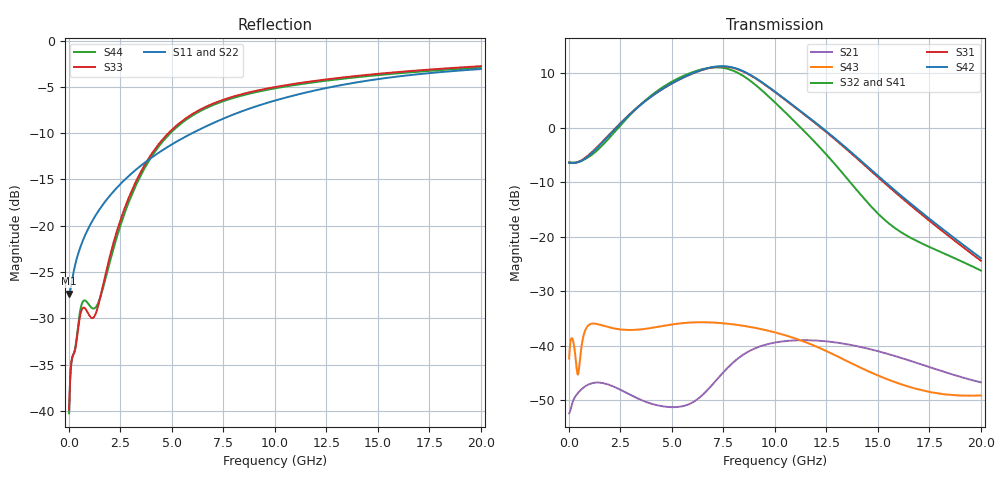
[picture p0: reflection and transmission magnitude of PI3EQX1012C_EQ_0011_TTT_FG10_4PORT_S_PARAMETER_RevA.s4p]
! NPort=4 DATA=2000 NOISE=0 GROUPDELAY=0 COMPLEX_DATAFORMAT=POLAR
! NumOfBlock=1 NumOfParam=0
! .MODEL Smodel S TSTONEFILE=PI3EQX1012C_EQ_0011_TTT_FG10_4PORT_S_PARAMETER_RevA.s4p TYPE=S
!  -- The above .MODEL line can be used for the S element in the netlist.
! The s parameter is extracted from the linear redriver, it is not bi-directional; only s(4,1)s(4,2) and s(3,1)s(3,2)
! should be the insertion loss
!Port definition:
!Port1 = input+
!Port2 = input-
!Port3 = output+
!Port4 = output-
# Hz S MA R  50
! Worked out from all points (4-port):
!   2000 points, 10 MHz to 20 GHz, reference 50 ohm
!   strongest paths, dB at 10 MHz, 5.01 GHz, 10.01 GHz, 15.01 GHz, 20 GHz:
!     S42: -6.4, 8.1, 6.6, -8.9, -24.0
!     S31: -6.4, 8.1, 6.5, -9.1, -24.4
!     S32: -6.4, 8.5, 4.6, -15.8, -26.2
!     S41: -6.4, 8.5, 4.7, -16.0, -26.6
!     S43: -42.4, -36.1, -37.6, -45.5, -49.2
!     S21: -52.4, -51.3, -39.5, -41.0, -46.8
!   lowest |S11| = -27.3 dB at 10 MHz (marker M1), VSWR 1.09, Z = 45.9 - j0.123 ohm
!   |S11| at or under -10 dB: start of sweep to 5.987 GHz
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1e7  0.04301 -178.2  0.002379 1.5  0.0008102 -0.5  0.0008039 -0.5
     0.002388 1.5  0.04109 -178.1  0.000927 -0.5  0.0009197 -0.5
     0.4783 -0.3  0.4774 179.8  0.01016 -4.0  0.007598 -25.7
     0.4769 179.8  0.4792 -0.3  0.007615 -25.8  0.009722 -4.1
4.07e9  0.2357 -124.4  0.002943 -0.6  0.0003837 -56.7  0.0003819 -57.1
        0.0029 -0.5  0.2393 -123.3  0.0004361 -57.4  0.0004341 -57.8
        1.973 -64.8  2.021 127.6  0.2497 -83.3  0.01353 33.9
        2.01 128.3  1.972 -63.1  0.01457 31.2  0.2417 -83.0
5.69e9  0.304 -123.9  0.002882 27.6  0.0002797 -58.5  0.0002786 -59.4
        0.002831 26.6  0.309 -123.2  0.0003171 -59.4  0.0003159 -60.3
        2.954 -129.7  3.059 62.7  0.3814 -98.9  0.0163 10.3
        3.069 62.9  2.968 -127.7  0.01616 7.6  0.3736 -98.7
7.04e9  0.36 -124.6  0.004731 47.3  0.0002393 -55.9  0.0002373 -57.3
        0.00454 47.5  0.3656 -124.1  0.0002699 -57.1  0.0002677 -58.4
        3.588 166.9  3.567 -0.9  0.4585 -109.5  0.01667 -10.6
        3.596 -1.1  3.613 169.0  0.01624 -11.9  0.4503 -109.3
8.29e9  0.4109 -126.0  0.008041 37.4  0.0002222 -54.1  0.0002191 -55.6
        0.007819 38.6  0.417 -125.6  0.000249 -55.4  0.0002455 -56.9
        3.375 101.7  3.117 -65.5  0.5096 -116.8  0.01573 -27.6
        3.155 -66.0  3.403 104.0  0.01536 -28.2  0.5011 -116.7
9.83e9  0.4681 -128.4  0.01064 12.6  0.0002119 -54.0  0.0002076 -55.6
        0.01049 13.8  0.4751 -128.0  0.0002356 -55.1  0.000231 -56.7
        2.24 29.7  1.829 -134.4  0.5564 -123.5  0.01378 -45.7
        1.856 -135.6  2.262 32.5  0.01346 -46.3  0.5476 -123.4
2e10  0.702 -144.6  0.004605 -65.1  0.0001466 -72.3  0.0001415 -73.8
      0.00459 -64.0  0.717 -144.3  0.0001626 -72.1  0.0001569 -73.7
      0.06004 109.2  0.04882 36.0  0.7272 -143.5  0.003565 -51.6
      0.04699 33.9  0.06341 113.9  0.003484 -49.0  0.7152 -143.3
